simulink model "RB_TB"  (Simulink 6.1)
settings: Solver=ode3  SolverMode=SingleTasking  StartTime=0  StopTime=1000  FixedStep=0.05  RelTol=1e-3
libraries: simulink x2
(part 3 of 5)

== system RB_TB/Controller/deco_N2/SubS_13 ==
  note: Pt of seconds
  note: Model: RB_TB/Controller/deco_N2/SubS_X
  Palv : Inport  Port=1  LatchInput=off
  Pamb_sea : Inport  Port=2  LatchInput=off
  Palv_INI : Inport  Port=3  LatchInput=off
  HT : Inport  Port=4  LatchInput=off
  BC1 : BusCreator  DialogController=Simulink.DDGSource_Bus
  Mux6 : Mux  Inputs=3
  Product1 : Product
  Sum2 : Sum  Inputs=|+-
  Sum3 : Sum  Inputs=++|
  fcn3 : Fcn  Expr=u(3)+u(2)/u(1)
  fcn5 : Fcn  Expr=log(2)/u(1)
  fcn6 : Fcn  Expr=1.005-u(1)^(-1/2)
  fcn7 : Fcn  Expr=2*u(1)^(-1/3)
  pr_PN2 : TransferFcn  Numerator=[1/60]  Denominator=[1 0]
  bus : Outport
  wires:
  Sum2/1 -> Product1/2
  Product1/1 -> pr_PN2/1
  fcn3/1 -> BC1/4  "M0"
  fcn6/1 -> Mux6/1, BC1/3  "N2_b"
  Mux6/1 -> fcn3/1
  fcn5/1 -> Product1/1, BC1/1  "N2_k"
  Palv/1 -> Sum2/1
  Pamb_sea/1 -> Mux6/2
  fcn7/1 -> Mux6/3  "N2_a"
  Sum3/1 -> BC1/2, Sum2/2  "Pt"
  Palv_INI/1 -> Sum3/1
  pr_PN2/1 -> Sum3/2
  BC1/1 -> bus/1
  HT/1 -> fcn7/1, fcn5/1, fcn6/1

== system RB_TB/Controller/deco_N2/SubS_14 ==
  note: Model: RB_TB/Controller/deco_N2/SubS_X
  note: Pt of seconds
  Palv : Inport  Port=1  LatchInput=off
  Pamb_sea : Inport  Port=2  LatchInput=off
  Palv_INI : Inport  Port=3  LatchInput=off
  HT : Inport  Port=4  LatchInput=off
  BC1 : BusCreator  DialogController=Simulink.DDGSource_Bus
  Mux6 : Mux  Inputs=3
  Product1 : Product
  Sum2 : Sum  Inputs=|+-
  Sum3 : Sum  Inputs=++|
  fcn3 : Fcn  Expr=u(3)+u(2)/u(1)
  fcn5 : Fcn  Expr=log(2)/u(1)
  fcn6 : Fcn  Expr=1.005-u(1)^(-1/2)
  fcn7 : Fcn  Expr=2*u(1)^(-1/3)
  pr_PN2 : TransferFcn  Numerator=[1/60]  Denominator=[1 0]
  bus : Outport
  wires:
  HT/1 -> fcn6/1, fcn5/1, fcn7/1
  BC1/1 -> bus/1
  pr_PN2/1 -> Sum3/2
  Palv_INI/1 -> Sum3/1
  Sum3/1 -> Sum2/2, BC1/2  "Pt"
  fcn7/1 -> Mux6/3  "N2_a"
  Pamb_sea/1 -> Mux6/2
  Palv/1 -> Sum2/1
  fcn5/1 -> BC1/1, Product1/1  "N2_k"
  Mux6/1 -> fcn3/1
  fcn6/1 -> BC1/3, Mux6/1  "N2_b"
  fcn3/1 -> BC1/4  "M0"
  Product1/1 -> pr_PN2/1
  Sum2/1 -> Product1/2

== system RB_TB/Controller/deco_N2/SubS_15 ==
  note: Pt of seconds
  note: Model: RB_TB/Controller/deco_N2/SubS_X
  Palv : Inport  Port=1  LatchInput=off
  Pamb_sea : Inport  Port=2  LatchInput=off
  Palv_INI : Inport  Port=3  LatchInput=off
  HT : Inport  Port=4  LatchInput=off
  BC1 : BusCreator  DialogController=Simulink.DDGSource_Bus
  Mux6 : Mux  Inputs=3
  Product1 : Product
  Sum2 : Sum  Inputs=|+-
  Sum3 : Sum  Inputs=++|
  fcn3 : Fcn  Expr=u(3)+u(2)/u(1)
  fcn5 : Fcn  Expr=log(2)/u(1)
  fcn6 : Fcn  Expr=1.005-u(1)^(-1/2)
  fcn7 : Fcn  Expr=2*u(1)^(-1/3)
  pr_PN2 : TransferFcn  Numerator=[1/60]  Denominator=[1 0]
  bus : Outport
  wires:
  Sum2/1 -> Product1/2
  Product1/1 -> pr_PN2/1
  fcn3/1 -> BC1/4  "M0"
  fcn6/1 -> Mux6/1, BC1/3  "N2_b"
  Mux6/1 -> fcn3/1
  fcn5/1 -> Product1/1, BC1/1  "N2_k"
  Palv/1 -> Sum2/1
  Pamb_sea/1 -> Mux6/2
  fcn7/1 -> Mux6/3  "N2_a"
  Sum3/1 -> BC1/2, Sum2/2  "Pt"
  Palv_INI/1 -> Sum3/1
  pr_PN2/1 -> Sum3/2
  BC1/1 -> bus/1
  HT/1 -> fcn7/1, fcn5/1, fcn6/1

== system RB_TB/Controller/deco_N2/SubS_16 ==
  note: Model: RB_TB/Controller/deco_N2/SubS_X
  note: Pt of seconds
  Palv : Inport  Port=1  LatchInput=off
  Pamb_sea : Inport  Port=2  LatchInput=off
  Palv_INI : Inport  Port=3  LatchInput=off
  HT : Inport  Port=4  LatchInput=off
  BC1 : BusCreator  DialogController=Simulink.DDGSource_Bus
  Mux6 : Mux  Inputs=3
  Product1 : Product
  Sum2 : Sum  Inputs=|+-
  Sum3 : Sum  Inputs=++|
  fcn3 : Fcn  Expr=u(3)+u(2)/u(1)
  fcn5 : Fcn  Expr=log(2)/u(1)
  fcn6 : Fcn  Expr=1.005-u(1)^(-1/2)
  fcn7 : Fcn  Expr=2*u(1)^(-1/3)
  pr_PN2 : TransferFcn  Numerator=[1/60]  Denominator=[1 0]
  bus : Outport
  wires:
  HT/1 -> fcn6/1, fcn5/1, fcn7/1
  BC1/1 -> bus/1
  pr_PN2/1 -> Sum3/2
  Palv_INI/1 -> Sum3/1
  Sum3/1 -> Sum2/2, BC1/2  "Pt"
  fcn7/1 -> Mux6/3  "N2_a"
  Pamb_sea/1 -> Mux6/2
  Palv/1 -> Sum2/1
  fcn5/1 -> BC1/1, Product1/1  "N2_k"
  Mux6/1 -> fcn3/1
  fcn6/1 -> BC1/3, Mux6/1  "N2_b"
  fcn3/1 -> BC1/4  "M0"
  Product1/1 -> pr_PN2/1
  Sum2/1 -> Product1/2

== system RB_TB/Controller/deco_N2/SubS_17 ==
  note: Pt of seconds
  note: Model: RB_TB/Controller/deco_N2/SubS_X
  Palv : Inport  Port=1  LatchInput=off
  Pamb_sea : Inport  Port=2  LatchInput=off
  Palv_INI : Inport  Port=3  LatchInput=off
  HT : Inport  Port=4  LatchInput=off
  BC1 : BusCreator  DialogController=Simulink.DDGSource_Bus
  Mux6 : Mux  Inputs=3
  Product1 : Product
  Sum2 : Sum  Inputs=|+-
  Sum3 : Sum  Inputs=++|
  fcn3 : Fcn  Expr=u(3)+u(2)/u(1)
  fcn5 : Fcn  Expr=log(2)/u(1)
  fcn6 : Fcn  Expr=1.005-u(1)^(-1/2)
  fcn7 : Fcn  Expr=2*u(1)^(-1/3)
  pr_PN2 : TransferFcn  Numerator=[1/60]  Denominator=[1 0]
  bus : Outport
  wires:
  Sum2/1 -> Product1/2
  Product1/1 -> pr_PN2/1
  fcn3/1 -> BC1/4  "M0"
  fcn6/1 -> Mux6/1, BC1/3  "N2_b"
  Mux6/1 -> fcn3/1
  fcn5/1 -> Product1/1, BC1/1  "N2_k"
  Palv/1 -> Sum2/1
  Pamb_sea/1 -> Mux6/2
  fcn7/1 -> Mux6/3  "N2_a"
  Sum3/1 -> BC1/2, Sum2/2  "Pt"
  Palv_INI/1 -> Sum3/1
  pr_PN2/1 -> Sum3/2
  BC1/1 -> bus/1
  HT/1 -> fcn7/1, fcn5/1, fcn6/1

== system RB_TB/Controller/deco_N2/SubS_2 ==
  note: Model: RB_TB/Controller/deco_N2/SubS_X
  note: Pt of seconds
  Palv : Inport  Port=1  LatchInput=off
  Pamb_sea : Inport  Port=2  LatchInput=off
  Palv_INI : Inport  Port=3  LatchInput=off
  HT : Inport  Port=4  LatchInput=off
  BC1 : BusCreator  DialogController=Simulink.DDGSource_Bus
  Mux6 : Mux  Inputs=3
  Product1 : Product
  Sum2 : Sum  Inputs=|+-
  Sum3 : Sum  Inputs=++|
  fcn3 : Fcn  Expr=u(3)+u(2)/u(1)
  fcn5 : Fcn  Expr=log(2)/u(1)
  fcn6 : Fcn  Expr=1.005-u(1)^(-1/2)
  fcn7 : Fcn  Expr=2*u(1)^(-1/3)
  pr_PN2 : TransferFcn  Numerator=[1/60]  Denominator=[1 0]
  bus : Outport
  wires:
  HT/1 -> fcn6/1, fcn5/1, fcn7/1
  BC1/1 -> bus/1
  pr_PN2/1 -> Sum3/2
  Palv_INI/1 -> Sum3/1
  Sum3/1 -> Sum2/2, BC1/2  "Pt"
  fcn7/1 -> Mux6/3  "N2_a"
  Pamb_sea/1 -> Mux6/2
  Palv/1 -> Sum2/1
  fcn5/1 -> BC1/1, Product1/1  "N2_k"
  Mux6/1 -> fcn3/1
  fcn6/1 -> BC1/3, Mux6/1  "N2_b"
  fcn3/1 -> BC1/4  "M0"
  Product1/1 -> pr_PN2/1
  Sum2/1 -> Product1/2

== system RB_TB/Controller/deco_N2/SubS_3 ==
  note: Pt of seconds
  note: Model: RB_TB/Controller/deco_N2/SubS_X
  Palv : Inport  Port=1  LatchInput=off
  Pamb_sea : Inport  Port=2  LatchInput=off
  Palv_INI : Inport  Port=3  LatchInput=off
  HT : Inport  Port=4  LatchInput=off
  BC1 : BusCreator  DialogController=Simulink.DDGSource_Bus
  Mux6 : Mux  Inputs=3
  Product1 : Product
  Sum2 : Sum  Inputs=|+-
  Sum3 : Sum  Inputs=++|
  fcn3 : Fcn  Expr=u(3)+u(2)/u(1)
  fcn5 : Fcn  Expr=log(2)/u(1)
  fcn6 : Fcn  Expr=1.005-u(1)^(-1/2)
  fcn7 : Fcn  Expr=2*u(1)^(-1/3)
  pr_PN2 : TransferFcn  Numerator=[1/60]  Denominator=[1 0]
  bus : Outport
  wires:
  Sum2/1 -> Product1/2
  Product1/1 -> pr_PN2/1
  fcn3/1 -> BC1/4  "M0"
  fcn6/1 -> Mux6/1, BC1/3  "N2_b"
  Mux6/1 -> fcn3/1
  fcn5/1 -> Product1/1, BC1/1  "N2_k"
  Palv/1 -> Sum2/1
  Pamb_sea/1 -> Mux6/2
  fcn7/1 -> Mux6/3  "N2_a"
  Sum3/1 -> BC1/2, Sum2/2  "Pt"
  Palv_INI/1 -> Sum3/1
  pr_PN2/1 -> Sum3/2
  BC1/1 -> bus/1
  HT/1 -> fcn7/1, fcn5/1, fcn6/1

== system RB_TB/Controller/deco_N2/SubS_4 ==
  note: Model: RB_TB/Controller/deco_N2/SubS_X
  note: Pt of seconds
  Palv : Inport  Port=1  LatchInput=off
  Pamb_sea : Inport  Port=2  LatchInput=off
  Palv_INI : Inport  Port=3  LatchInput=off
  HT : Inport  Port=4  LatchInput=off
  BC1 : BusCreator  DialogController=Simulink.DDGSource_Bus
  Mux6 : Mux  Inputs=3
  Product1 : Product
  Sum2 : Sum  Inputs=|+-
  Sum3 : Sum  Inputs=++|
  fcn3 : Fcn  Expr=u(3)+u(2)/u(1)
  fcn5 : Fcn  Expr=log(2)/u(1)
  fcn6 : Fcn  Expr=1.005-u(1)^(-1/2)
  fcn7 : Fcn  Expr=2*u(1)^(-1/3)
  pr_PN2 : TransferFcn  Numerator=[1/60]  Denominator=[1 0]
  bus : Outport
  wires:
  HT/1 -> fcn6/1, fcn5/1, fcn7/1
  BC1/1 -> bus/1
  pr_PN2/1 -> Sum3/2
  Palv_INI/1 -> Sum3/1
  Sum3/1 -> Sum2/2, BC1/2  "Pt"
  fcn7/1 -> Mux6/3  "N2_a"
  Pamb_sea/1 -> Mux6/2
  Palv/1 -> Sum2/1
  fcn5/1 -> BC1/1, Product1/1  "N2_k"
  Mux6/1 -> fcn3/1
  fcn6/1 -> BC1/3, Mux6/1  "N2_b"
  fcn3/1 -> BC1/4  "M0"
  Product1/1 -> pr_PN2/1
  Sum2/1 -> Product1/2

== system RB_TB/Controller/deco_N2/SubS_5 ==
  note: Pt of seconds
  note: Model: RB_TB/Controller/deco_N2/SubS_X
  Palv : Inport  Port=1  LatchInput=off
  Pamb_sea : Inport  Port=2  LatchInput=off
  Palv_INI : Inport  Port=3  LatchInput=off
  HT : Inport  Port=4  LatchInput=off
  BC1 : BusCreator  DialogController=Simulink.DDGSource_Bus
  Mux6 : Mux  Inputs=3
  Product1 : Product
  Sum2 : Sum  Inputs=|+-
  Sum3 : Sum  Inputs=++|
  fcn3 : Fcn  Expr=u(3)+u(2)/u(1)
  fcn5 : Fcn  Expr=log(2)/u(1)
  fcn6 : Fcn  Expr=1.005-u(1)^(-1/2)
  fcn7 : Fcn  Expr=2*u(1)^(-1/3)
  pr_PN2 : TransferFcn  Numerator=[1/60]  Denominator=[1 0]
  bus : Outport
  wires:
  Sum2/1 -> Product1/2
  Product1/1 -> pr_PN2/1
  fcn3/1 -> BC1/4  "M0"
  fcn6/1 -> Mux6/1, BC1/3  "N2_b"
  Mux6/1 -> fcn3/1
  fcn5/1 -> Product1/1, BC1/1  "N2_k"
  Palv/1 -> Sum2/1
  Pamb_sea/1 -> Mux6/2
  fcn7/1 -> Mux6/3  "N2_a"
  Sum3/1 -> BC1/2, Sum2/2  "Pt"
  Palv_INI/1 -> Sum3/1
  pr_PN2/1 -> Sum3/2
  BC1/1 -> bus/1
  HT/1 -> fcn7/1, fcn5/1, fcn6/1

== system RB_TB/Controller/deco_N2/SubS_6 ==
  note: Model: RB_TB/Controller/deco_N2/SubS_X
  note: Pt of seconds
  Palv : Inport  Port=1  LatchInput=off
  Pamb_sea : Inport  Port=2  LatchInput=off
  Palv_INI : Inport  Port=3  LatchInput=off
  HT : Inport  Port=4  LatchInput=off
  BC1 : BusCreator  DialogController=Simulink.DDGSource_Bus
  Mux6 : Mux  Inputs=3
  Product1 : Product
  Sum2 : Sum  Inputs=|+-
  Sum3 : Sum  Inputs=++|
  fcn3 : Fcn  Expr=u(3)+u(2)/u(1)
  fcn5 : Fcn  Expr=log(2)/u(1)
  fcn6 : Fcn  Expr=1.005-u(1)^(-1/2)
  fcn7 : Fcn  Expr=2*u(1)^(-1/3)
  pr_PN2 : TransferFcn  Numerator=[1/60]  Denominator=[1 0]
  bus : Outport
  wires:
  HT/1 -> fcn6/1, fcn5/1, fcn7/1
  BC1/1 -> bus/1
  pr_PN2/1 -> Sum3/2
  Palv_INI/1 -> Sum3/1
  Sum3/1 -> Sum2/2, BC1/2  "Pt"
  fcn7/1 -> Mux6/3  "N2_a"
  Pamb_sea/1 -> Mux6/2
  Palv/1 -> Sum2/1
  fcn5/1 -> BC1/1, Product1/1  "N2_k"
  Mux6/1 -> fcn3/1
  fcn6/1 -> BC1/3, Mux6/1  "N2_b"
  fcn3/1 -> BC1/4  "M0"
  Product1/1 -> pr_PN2/1
  Sum2/1 -> Product1/2

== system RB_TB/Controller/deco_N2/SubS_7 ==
  note: Pt of seconds
  note: Model: RB_TB/Controller/deco_N2/SubS_X
  Palv : Inport  Port=1  LatchInput=off
  Pamb_sea : Inport  Port=2  LatchInput=off
  Palv_INI : Inport  Port=3  LatchInput=off
  HT : Inport  Port=4  LatchInput=off
  BC1 : BusCreator  DialogController=Simulink.DDGSource_Bus
  Mux6 : Mux  Inputs=3
  Product1 : Product
  Sum2 : Sum  Inputs=|+-
  Sum3 : Sum  Inputs=++|
  fcn3 : Fcn  Expr=u(3)+u(2)/u(1)
  fcn5 : Fcn  Expr=log(2)/u(1)
  fcn6 : Fcn  Expr=1.005-u(1)^(-1/2)
  fcn7 : Fcn  Expr=2*u(1)^(-1/3)
  pr_PN2 : TransferFcn  Numerator=[1/60]  Denominator=[1 0]
  bus : Outport
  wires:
  Sum2/1 -> Product1/2
  Product1/1 -> pr_PN2/1
  fcn3/1 -> BC1/4  "M0"
  fcn6/1 -> Mux6/1, BC1/3  "N2_b"
  Mux6/1 -> fcn3/1
  fcn5/1 -> Product1/1, BC1/1  "N2_k"
  Palv/1 -> Sum2/1
  Pamb_sea/1 -> Mux6/2
  fcn7/1 -> Mux6/3  "N2_a"
  Sum3/1 -> BC1/2, Sum2/2  "Pt"
  Palv_INI/1 -> Sum3/1
  pr_PN2/1 -> Sum3/2
  BC1/1 -> bus/1
  HT/1 -> fcn7/1, fcn5/1, fcn6/1

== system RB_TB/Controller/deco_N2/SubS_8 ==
  note: Model: RB_TB/Controller/deco_N2/SubS_X
  note: Pt of seconds
  Palv : Inport  Port=1  LatchInput=off
  Pamb_sea : Inport  Port=2  LatchInput=off
  Palv_INI : Inport  Port=3  LatchInput=off
  HT : Inport  Port=4  LatchInput=off
  BC1 : BusCreator  DialogController=Simulink.DDGSource_Bus
  Mux6 : Mux  Inputs=3
  Product1 : Product
  Sum2 : Sum  Inputs=|+-
  Sum3 : Sum  Inputs=++|
  fcn3 : Fcn  Expr=u(3)+u(2)/u(1)
  fcn5 : Fcn  Expr=log(2)/u(1)
  fcn6 : Fcn  Expr=1.005-u(1)^(-1/2)
  fcn7 : Fcn  Expr=2*u(1)^(-1/3)
  pr_PN2 : TransferFcn  Numerator=[1/60]  Denominator=[1 0]
  bus : Outport
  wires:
  HT/1 -> fcn6/1, fcn5/1, fcn7/1
  BC1/1 -> bus/1
  pr_PN2/1 -> Sum3/2
  Palv_INI/1 -> Sum3/1
  Sum3/1 -> Sum2/2, BC1/2  "Pt"
  fcn7/1 -> Mux6/3  "N2_a"
  Pamb_sea/1 -> Mux6/2
  Palv/1 -> Sum2/1
  fcn5/1 -> BC1/1, Product1/1  "N2_k"
  Mux6/1 -> fcn3/1
  fcn6/1 -> BC1/3, Mux6/1  "N2_b"
  fcn3/1 -> BC1/4  "M0"
  Product1/1 -> pr_PN2/1
  Sum2/1 -> Product1/2

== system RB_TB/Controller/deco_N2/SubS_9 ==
  note: Pt of seconds
  note: Model: RB_TB/Controller/deco_N2/SubS_X
  Palv : Inport  Port=1  LatchInput=off
  Pamb_sea : Inport  Port=2  LatchInput=off
  Palv_INI : Inport  Port=3  LatchInput=off
  HT : Inport  Port=4  LatchInput=off
  BC1 : BusCreator  DialogController=Simulink.DDGSource_Bus
  Mux6 : Mux  Inputs=3
  Product1 : Product
  Sum2 : Sum  Inputs=|+-
  Sum3 : Sum  Inputs=++|
  fcn3 : Fcn  Expr=u(3)+u(2)/u(1)
  fcn5 : Fcn  Expr=log(2)/u(1)
  fcn6 : Fcn  Expr=1.005-u(1)^(-1/2)
  fcn7 : Fcn  Expr=2*u(1)^(-1/3)
  pr_PN2 : TransferFcn  Numerator=[1/60]  Denominator=[1 0]
  bus : Outport
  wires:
  Sum2/1 -> Product1/2
  Product1/1 -> pr_PN2/1
  fcn3/1 -> BC1/4  "M0"
  fcn6/1 -> Mux6/1, BC1/3  "N2_b"
  Mux6/1 -> fcn3/1
  fcn5/1 -> Product1/1, BC1/1  "N2_k"
  Palv/1 -> Sum2/1
  Pamb_sea/1 -> Mux6/2
  fcn7/1 -> Mux6/3  "N2_a"
  Sum3/1 -> BC1/2, Sum2/2  "Pt"
  Palv_INI/1 -> Sum3/1
  pr_PN2/1 -> Sum3/2
  BC1/1 -> bus/1
  HT/1 -> fcn7/1, fcn5/1, fcn6/1

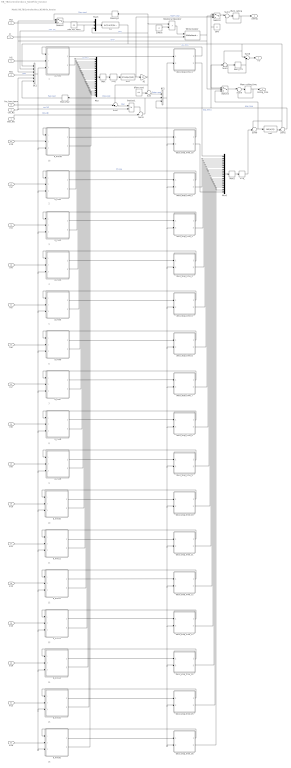
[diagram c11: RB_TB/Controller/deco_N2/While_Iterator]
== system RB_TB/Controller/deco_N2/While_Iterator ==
  note: 1
  note: 2
  note: 3
  note: 4
  note: 5
  note: 6
  note: 7
  note: 8
  note: 9
  note: 10
  note: 11
  note: 12
  note: 13
  note: 14
  note: 15
  note: 16
  note: Model: RB_TB/Controller/deco_N2/While_Iterator
  note: 1b
  cnc_N2 : Inport  Port=1  LatchInput=off
  Psw : Inport  Port=2  LatchInput=off
  IC : Inport  Port=3  LatchInput=off
  Palv : Inport  Port=4  LatchInput=off
  In1 : Inport  Port=5  LatchInput=off
  In2 : Inport  Port=6  LatchInput=off
  Palv_INI : Inport  Port=7  LatchInput=off
  fnc_hum_temp : Inport  Port=8  LatchInput=off
  In3 : Inport  Port=9  LatchInput=off
  In4 : Inport  Port=10  LatchInput=off
  In5 : Inport  Port=11  LatchInput=off
  In6 : Inport  Port=12  LatchInput=off
  In7 : Inport  Port=13  LatchInput=off
  In8 : Inport  Port=14  LatchInput=off
  In9 : Inport  Port=15  LatchInput=off
  In10 : Inport  Port=16  LatchInput=off
  In11 : Inport  Port=17  LatchInput=off
  In12 : Inport  Port=18  LatchInput=off
  In13 : Inport  Port=19  LatchInput=off
  In14 : Inport  Port=20  LatchInput=off
  In15 : Inport  Port=21  LatchInput=off
  In16 : Inport  Port=22  LatchInput=off
  In1b : Inport  Port=23  LatchInput=off
  >=0 : DeadZone  LowerValue=-1000  UpperValue=0
  >=0_ : DeadZone  LowerValue=-inf  UpperValue=0
  BC1 : BusCreator  DialogController=Simulink.DDGSource_Bus  Inputs=6
  BC2 : BusCreator  DialogController=Simulink.DDGSource_Bus  Inputs=3
  K1 : Gain  Gain=0.1
  Max : MinMax  Function=max
  Max1 : MinMax  Function=max
  Mem_Palv : Memory  Orientation=left  InheritSampleTime=on
  Mem_TTS : Memory  InheritSampleTime=on
  Mem_ceiling : Memory  InheritSampleTime=on
  Mem_ceiling_time : Memory  InheritSampleTime=on
  Memory2 : Memory  Orientation=left  InheritSampleTime=on
  Mux : Mux  Inputs=17
  Mux1 : Mux  Inputs=17
  Mux3 : Mux  Inputs=3
  Product1 : Product
  Relational Operator : RelationalOperator  Operator=>  LogicOutDataTypeMode=Boolean
  Suface : Constant  Value=0
  Sum : Sum  Inputs=+-|
  Sum1 : Sum  Inputs=|++
  Sum2 : Sum  Inputs=-+|
  Sum3 : Sum  Inputs=+++
  Sum4 : Sum  Inputs=|++
  Sum5 : Sum
  Sum6 : Sum  Inputs=++|
  Sum7 : Sum  Inputs=++|
  Sum8 : Sum
  Switch1 : Switch  Threshold=2
  Switch2 : Switch  Threshold=2
  Switch3 : Switch  Threshold=2
  While Iterator : WhileIterator  MaxIters=100  ShowIterationPort=on
  dPsw_next : Constant  Value=0.3
  d_min1 : Subsystem
  d_min10 : Subsystem
  d_min11 : Subsystem
  d_min12 : Subsystem
  d_min13 : Subsystem
  d_min14 : Subsystem
  d_min15 : Subsystem
  d_min16 : Subsystem
  d_min1b : Subsystem
  d_min2 : Subsystem
  d_min3 : Subsystem
  d_min4 : Subsystem
  d_min5 : Subsystem
  d_min6 : Subsystem
  d_min7 : Subsystem
  d_min8 : Subsystem
  d_min9 : Subsystem
  deco_stop_time_1 : Subsystem
  deco_stop_time_10 : Subsystem
  deco_stop_time_11 : Subsystem
  deco_stop_time_12 : Subsystem
  deco_stop_time_13 : Subsystem
  deco_stop_time_14 : Subsystem
  deco_stop_time_15 : Subsystem
  deco_stop_time_16 : Subsystem
  deco_stop_time_1b : Subsystem
  deco_stop_time_2 : Subsystem
  deco_stop_time_3 : Subsystem
  deco_stop_time_4 : Subsystem
  deco_stop_time_5 : Subsystem
  deco_stop_time_6 : Subsystem
  deco_stop_time_7 : Subsystem
  deco_stop_time_8 : Subsystem
  deco_stop_time_9 : Subsystem
  fcn : Fcn  Expr=(u(1)-u(3))/u(2)
  fcn1 : Fcn  Expr=ceil(u(1))
  fcn2 : Fcn  Expr=3*ceil(u(1)/3)
  rate_asc_deco : Constant  Value=0.9
  zero : Constant  Orientation=left  Value=0
  TTS : Outport
  ceiling : Outport  Port=2
  ceiling_time : Outport  Port=3
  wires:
  IC/1 -> While Iterator/2
  Mux/1 -> Max/1
  fcn2/1 -> K1/1, Switch1/3  "Depth_stop"
  Max/1 -> >=0/1
  >=0/1 -> fcn2/1
  rate_asc_deco/1 -> Mux3/2, BC1/2  "rate_asc"
  K1/1 -> Sum7/1, Sum/1, Mux3/3, Memory2/1, Relational Operator/1  "Psw"
  Max1/1 -> >=0_/1
  Mux3/1 -> fcn/1
  deco_stop_time_1/2(deco_stop_time) -> Mux1/1  "stop_time_i"
  fcn/1 -> Sum8/1, Sum3/1, Sum2/1, Sum6/1, BC1/1  "asc_time"
  d_min1/2(d_min) -> Mux/1  "d_min_i"
  Mem_TTS/1 -> Sum8/2, Sum3/3
  Sum3/1 -> Mem_TTS/1
  cnc_N2/1 -> Product1/2, BC1/5  "cnc_N2"
  Product1/1 -> Sum5/1
  Palv_INI/1 -> Sum5/2  "Palv_INI"
  fnc_hum_temp/1 -> Sum7/2
  Sum5/1 -> Mem_Palv/1, BC2/2  "Palv_next"
  Sum7/1 -> Product1/1  "Psw'"
  d_min1/1(bus1) -> deco_stop_time_1/1(bus1)
  d_min2/1(bus1) -> deco_stop_time_2/1(bus1)
  d_min2/2(d_min) -> Mux/2
  In1/1 -> d_min1/2(In1)
  Mem_Palv/1 -> BC1/6  "Palv_next"
  Psw/1 -> Switch2/3
  Switch2/1 -> Mux3/1
  Memory2/1 -> Switch2/1  "Psw_nwxt"
  deco_stop_time_1/1(Pt_new) -> d_min1/1(Pt_new)
  dPsw_next/1 -> Sum/2
  Sum/1 -> BC2/1  "Pstop_next"
  deco_stop_time_2/1(Pt_new) -> d_min2/1(Pt_new)  "Pt_new"
  Sum2/1 -> BC2/3, Sum3/2  "stop_time"
  fcn1/1 -> Sum2/2
  Sum6/1 -> fcn1/1, Switch3/3
  >=0_/1 -> Sum6/2
  Suface/1 -> Relational Operator/2
  Relational Operator/1 -> While Iterator/1
  Sum1/1 -> Mem_ceiling/1
  Mem_ceiling/1 -> ceiling/1, Sum1/2
  Switch1/1 -> Sum1/1
  Mem_ceiling_time/1 -> ceiling_time/1, Sum4/2
  Sum8/1 -> TTS/1
  Palv/1 -> BC1/4  "Palv"
  BC1/1 -> d_min1/3(In2), d_min15/3(In2), d_min16/3(In2), d_min14/3(In2), d_min13/3(In2), d_min12/3(In2), d_min11/3(In2), d_min10/3(In2), d_min9/3(In2), d_min8/3(In2), d_min7/3(In2), d_min6/3(In2), d_min5/3(In2), d_min4/3(In2), d_min3/3(In2), d_min2/3(In2), d_min1b/3(In2)
  In2/1 -> d_min2/2(In1)
  BC2/1 -> deco_stop_time_1/2(bus2), deco_stop_time_15/2(bus2), deco_stop_time_16/2(bus2), deco_stop_time_14/2(bus2), deco_stop_time_13/2(bus2), deco_stop_time_12/2(bus2), deco_stop_time_11/2(bus2), deco_stop_time_10/2(bus2), deco_stop_time_9/2(bus2), deco_stop_time_8/2(bus2), deco_stop_time_7/2(bus2), deco_stop_time_6/2(bus2), deco_stop_time_5/2(bus2), deco_stop_time_4/2(bus2), deco_stop_time_3/2(bus2), deco_stop_time_2/2(bus2), deco_stop_time_1b/2(bus2)
  zero/1 -> Switch1/1, Switch3/1
  While Iterator/1 -> BC1/3, Switch2/2, Switch3/2, Switch1/2  "while"
  d_min3/1(bus1) -> deco_stop_time_3/1(bus1)
  deco_stop_time_3/1(Pt_new) -> d_min3/1(Pt_new)
  In3/1 -> d_min3/2(In1)
  In4/1 -> d_min4/2(In1)
  deco_stop_time_4/1(Pt_new) -> d_min4/1(Pt_new)
  d_min4/1(bus1) -> deco_stop_time_4/1(bus1)
  d_min5/1(bus1) -> deco_stop_time_5/1(bus1)
  deco_stop_time_5/1(Pt_new) -> d_min5/1(Pt_new)
  In5/1 -> d_min5/2(In1)
  In6/1 -> d_min6/2(In1)
  deco_stop_time_6/1(Pt_new) -> d_min6/1(Pt_new)
  d_min6/1(bus1) -> deco_stop_time_6/1(bus1)
  d_min7/1(bus1) -> deco_stop_time_7/1(bus1)
  deco_stop_time_7/1(Pt_new) -> d_min7/1(Pt_new)
  In7/1 -> d_min7/2(In1)
  In8/1 -> d_min8/2(In1)
  deco_stop_time_8/1(Pt_new) -> d_min8/1(Pt_new)
  d_min8/1(bus1) -> deco_stop_time_8/1(bus1)
  d_min9/1(bus1) -> deco_stop_time_9/1(bus1)
  deco_stop_time_9/1(Pt_new) -> d_min9/1(Pt_new)
  In9/1 -> d_min9/2(In1)
  In10/1 -> d_min10/2(In1)
  deco_stop_time_10/1(Pt_new) -> d_min10/1(Pt_new)
  d_min10/1(bus1) -> deco_stop_time_10/1(bus1)
  d_min11/1(bus1) -> deco_stop_time_11/1(bus1)
  deco_stop_time_11/1(Pt_new) -> d_min11/1(Pt_new)
  In11/1 -> d_min11/2(In1)
  In12/1 -> d_min12/2(In1)
  deco_stop_time_12/1(Pt_new) -> d_min12/1(Pt_new)
  d_min12/1(bus1) -> deco_stop_time_12/1(bus1)
  d_min13/1(bus1) -> deco_stop_time_13/1(bus1)
  deco_stop_time_13/1(Pt_new) -> d_min13/1(Pt_new)
  In13/1 -> d_min13/2(In1)
  In14/1 -> d_min14/2(In1)
  deco_stop_time_14/1(Pt_new) -> d_min14/1(Pt_new)
  d_min14/1(bus1) -> deco_stop_time_14/1(bus1)
  d_min15/1(bus1) -> deco_stop_time_15/1(bus1)
  deco_stop_time_15/1(Pt_new) -> d_min15/1(Pt_new)
  In15/1 -> d_min15/2(In1)
  In16/1 -> d_min16/2(In1)
  deco_stop_time_16/1(Pt_new) -> d_min16/1(Pt_new)
  d_min16/1(bus1) -> deco_stop_time_16/1(bus1)
  Mux1/1 -> Max1/1
  deco_stop_time_2/2(deco_stop_time) -> Mux1/2
  d_min3/2(d_min) -> Mux/3
  d_min4/2(d_min) -> Mux/4
  d_min5/2(d_min) -> Mux/5
  d_min6/2(d_min) -> Mux/6
  d_min7/2(d_min) -> Mux/7
  d_min8/2(d_min) -> Mux/8
  d_min9/2(d_min) -> Mux/9
  d_min10/2(d_min) -> Mux/10
  d_min11/2(d_min) -> Mux/11
  d_min12/2(d_min) -> Mux/12
  d_min13/2(d_min) -> Mux/13
  d_min14/2(d_min) -> Mux/14
  d_min15/2(d_min) -> Mux/15
  d_min16/2(d_min) -> Mux/16
  deco_stop_time_3/2(deco_stop_time) -> Mux1/3
  deco_stop_time_4/2(deco_stop_time) -> Mux1/4
  deco_stop_time_5/2(deco_stop_time) -> Mux1/5
  deco_stop_time_6/2(deco_stop_time) -> Mux1/6
  deco_stop_time_7/2(deco_stop_time) -> Mux1/7
  deco_stop_time_8/2(deco_stop_time) -> Mux1/8
  deco_stop_time_9/2(deco_stop_time) -> Mux1/9
  deco_stop_time_10/2(deco_stop_time) -> Mux1/10
  deco_stop_time_11/2(deco_stop_time) -> Mux1/11
  deco_stop_time_12/2(deco_stop_time) -> Mux1/12
  deco_stop_time_13/2(deco_stop_time) -> Mux1/13
  deco_stop_time_14/2(deco_stop_time) -> Mux1/14
  deco_stop_time_15/2(deco_stop_time) -> Mux1/15
  deco_stop_time_16/2(deco_stop_time) -> Mux1/16
  Sum4/1 -> Mem_ceiling_time/1
  Switch3/1 -> Sum4/1
  d_min1b/1(bus1) -> deco_stop_time_1b/1(bus1)
  deco_stop_time_1b/1(Pt_new) -> d_min1b/1(Pt_new)
  In1b/1 -> d_min1b/2(In1)
  d_min1b/2(d_min) -> Mux/17
  deco_stop_time_1b/2(deco_stop_time) -> Mux1/17

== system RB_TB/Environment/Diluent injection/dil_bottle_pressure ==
  note: Model: RB_TB/Environment/Diluent injection/pr_dil_bottle
  gas_mix : Inport  Port=1  LatchInput=off
  F_D : Inport  Port=2  LatchInput=off
  Fcn : Fcn  Expr=u(1)/u(2)
  Multiport Switch : MultiPortSwitch  Inputs=3
  Multiport Switch1 : MultiPortSwitch  Inputs=3
  Multiport Switch2 : MultiPortSwitch  Inputs=3
  Mux : Mux  Inputs=2
  Product : Product
  Product2 : Product
  Product3 : Product
  Sum : Sum  Inputs=+-
  Sum2 : Sum  Inputs=+-
  Sum3 : Sum  Inputs=+-
  Sw1 : MultiPortSwitch  Inputs=3
  Sw3 : MultiPortSwitch  Inputs=3
  Sw4 : MultiPortSwitch  Inputs=3
  integral1 : Integrator
  integral2 : Integrator
  integral3 : Integrator
  pr_dil_bottle1_ini : Constant  Value=230
  pr_dil_bottle2_ini : Constant  Value=230
  pr_dil_bottle3_ini : Constant  Value=230
  size_dil_bottle1 : Constant  Value=3
  size_dil_bottle2 : Constant  Value=3
  size_dil_bottle3 : Constant  Value=3
  zero : Constant  Value=0
  O2 : Outport
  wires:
  Product/1 -> Sum/1  "vol_dil_bottle1_ini"
  integral1/1 -> Sum/2
  gas_mix/1 -> Sw4/1, Sw3/1, Sw1/1, Multiport Switch/1, Multiport Switch1/1, Multiport Switch2/1
  Sum/1 -> Multiport Switch/2
  Multiport Switch/1 -> Mux/1  "vol_dil_bottle"
  Sw1/1 -> integral1/1
  zero/1 -> Sw4/4, Sw3/2, Sw3/3, Sw4/2, Sw1/3, Sw1/4
  F_D/1 -> Sw1/2, Sw4/3, Sw3/4
  Mux/1 -> Fcn/1
  Fcn/1 -> O2/1  "pr_dil_bottle"
  size_dil_bottle1/1 -> Product/1, Multiport Switch1/2
  pr_dil_bottle1_ini/1 -> Product/2, Multiport Switch2/2
  Product2/1 -> Sum2/1  "vol_dil_bottle2_ini"
  integral2/1 -> Sum2/2
  Sw4/1 -> integral2/1
  size_dil_bottle2/1 -> Product2/1, Multiport Switch1/3
  pr_dil_bottle2_ini/1 -> Product2/2, Multiport Switch2/3
  Product3/1 -> Sum3/1  "vol_dil_bottle3_ini"
  integral3/1 -> Sum3/2
  Sw3/1 -> integral3/1
  size_dil_bottle3/1 -> Product3/1, Multiport Switch1/4
  pr_dil_bottle3_ini/1 -> Product3/2, Multiport Switch2/4
  Sum2/1 -> Multiport Switch/3
  Sum3/1 -> Multiport Switch/4
  Multiport Switch1/1 -> Mux/2  "size_dil_bottle"
  Multiport Switch2/1 -> [pr_dil_bottle_ini]

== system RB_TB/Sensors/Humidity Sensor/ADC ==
  note: Model: RB_TB/Sensors/Humidity_sensor/ADC
  note: This subsystem models a typical 16-bit analog-to-digital converter having an input range of 0-5 volts
  voltage : Inport  Port=1  LatchInput=off
  limit : Saturate  UpperLimit=65535  LowerLimit=0
  quantize : Quantizer  QuantizationInterval=1
  scale : Gain  Gain=65536/5
  pcm : Outport
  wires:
  limit/1 -> pcm/1
  scale/1 -> quantize/1
  quantize/1 -> limit/1
  voltage/1 -> scale/1

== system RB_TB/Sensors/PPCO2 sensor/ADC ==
  note: This subsystem models a typical 16-bit analog-to-digital converter having an input range of 0-5 volts
  note: Model: RB_TB/Sensors/PPCO2 sensor/ADC
  voltage : Inport  Port=1  LatchInput=off
  limit : Saturate  UpperLimit=65535  LowerLimit=0
  quantize : Quantizer  QuantizationInterval=1
  scale : Gain  Gain=65536/5
  pcm : Outport
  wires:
  voltage/1 -> scale/1
  quantize/1 -> limit/1
  scale/1 -> quantize/1
  limit/1 -> pcm/1

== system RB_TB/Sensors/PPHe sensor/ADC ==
  note: Model: RB_TB/Sensors/PPO2 sensor/ADC
  note: This subsystem models a typical 16-bit analog-to-digital converter having an input range of 0-5 volts
  voltage : Inport  Port=1  LatchInput=off
  limit : Saturate  UpperLimit=65535  LowerLimit=0
  quantize : Quantizer  QuantizationInterval=1
  scale : Gain  Gain=65536/5
  pcm : Outport
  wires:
  voltage/1 -> scale/1
  quantize/1 -> limit/1
  scale/1 -> quantize/1
  limit/1 -> pcm/1

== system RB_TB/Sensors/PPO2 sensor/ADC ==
  note: This subsystem models a typical 16-bit analog-to-digital converter having an input range of 0-5 volts
  note: Model: RB_TB/Sensors/PPO2 sensor/ADC
  voltage : Inport  Port=1  LatchInput=off
  limit : Saturate  UpperLimit=65535  LowerLimit=0
  quantize : Quantizer  QuantizationInterval=1
  scale : Gain  Gain=65536/5
  pcm : Outport
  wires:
  limit/1 -> pcm/1
  scale/1 -> quantize/1
  quantize/1 -> limit/1
  voltage/1 -> scale/1

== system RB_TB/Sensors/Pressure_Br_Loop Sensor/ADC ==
  note: This subsystem models a typical 15-bit analog-to-digital converter having an input range of 0-3 volts
  note: Model: RB_TB/Sensors/Pressure_ambient Sensor/ADC
  voltage : Inport  Port=1  LatchInput=off
  limit : Saturate  UpperLimit=2^15  LowerLimit=0
  quantize : Quantizer  QuantizationInterval=1
  scale : Gain  Gain=2^15/3
  pcm : Outport
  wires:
  voltage/1 -> scale/1
  quantize/1 -> limit/1
  scale/1 -> quantize/1
  limit/1 -> pcm/1

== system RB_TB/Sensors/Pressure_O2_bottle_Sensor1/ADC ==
  note: Model: RB_TB/Sensors/Pressure_ambient Sensor/ADC
  note: This subsystem models a typical 15-bit analog-to-digital converter having an input range of 0-3 volts
  voltage : Inport  Port=1  LatchInput=off
  limit : Saturate  UpperLimit=2^15  LowerLimit=0
  quantize : Quantizer  QuantizationInterval=1
  scale : Gain  Gain=2^15/3
  pcm : Outport
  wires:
  limit/1 -> pcm/1
  scale/1 -> quantize/1
  quantize/1 -> limit/1
  voltage/1 -> scale/1

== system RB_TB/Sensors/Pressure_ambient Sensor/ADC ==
  note: Model: RB_TB/Sensors/Pressure_ambient Sensor/ADC
  note: This subsystem models a typical 15-bit analog-to-digital converter having an input range of 0-3 volts
  voltage : Inport  Port=1  LatchInput=off
  limit : Saturate  UpperLimit=2^15  LowerLimit=0
  quantize : Quantizer  QuantizationInterval=1
  scale : Gain  Gain=2^15/3
  pcm : Outport
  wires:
  limit/1 -> pcm/1
  scale/1 -> quantize/1
  quantize/1 -> limit/1
  voltage/1 -> scale/1

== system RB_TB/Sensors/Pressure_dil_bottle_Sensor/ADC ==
  note: This subsystem models a typical 15-bit analog-to-digital converter having an input range of 0-3 volts
  note: Model: RB_TB/Sensors/Pressure_ambient Sensor/ADC
  voltage : Inport  Port=1  LatchInput=off
  limit : Saturate  UpperLimit=2^15  LowerLimit=0
  quantize : Quantizer  QuantizationInterval=1
  scale : Gain  Gain=2^15/3
  pcm : Outport
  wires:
  voltage/1 -> scale/1
  quantize/1 -> limit/1
  scale/1 -> quantize/1
  limit/1 -> pcm/1

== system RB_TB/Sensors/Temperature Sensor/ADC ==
  note: This subsystem models a typical 16-bit analog-to-digital converter having an input range of 0-5 volts
  note: Model: RB_TB/Sensors/temperature_sensor/ADC
  voltage : Inport  Port=1  LatchInput=off
  limit : Saturate  UpperLimit=65535  LowerLimit=0
  quantize : Quantizer  QuantizationInterval=1
  scale : Gain  Gain=65536/5
  pcm : Outport
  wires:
  voltage/1 -> scale/1
  quantize/1 -> limit/1
  scale/1 -> quantize/1
  limit/1 -> pcm/1

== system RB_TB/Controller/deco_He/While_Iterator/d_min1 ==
  note: Model: RB_TB/Controller/deco_He/While_Iterator/d_minX
  Pt_new : Inport  Port=1  LatchInput=off
  In1 : Inport  Port=2  LatchInput=off
  In2 : Inport  Port=3  LatchInput=off
  BC : BusCreator  DialogController=Simulink.DDGSource_Bus
  BS1 : BusSelector  DialogController=Simulink.DDGSource_Bus  OutputSignals=He_b,M0,He_k,Pt
  BS2 : BusSelector  DialogController=Simulink.DDGSource_Bus  OutputSignals=rate_asc,asc_time,while,cnc_He,Palv_next,Palv
  Mux2 : Mux  Inputs=6
  Product2 : Product
  Sum1 : Sum  Inputs=-+|
  Switch : Switch  Threshold=2
  Switch1 : Switch  Threshold=2
  fnc : Fcn  Expr=u(6)-u(5)*u(2)*(u(3)-1/u(1))-(u(6)-u(4)+u(5)*u(2)/u(1))*exp(-u(1)*u(3))
  prod : Gain  Gain=10
  bus1 : Outport
  d_min : Outport  Port=2
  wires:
  BS2/1 -> Mux2/2  "<rate_asc>"
  In2/1 -> BS2/1
  BS2/5 -> Switch1/1  "<Palv_next>"
  BS2/3 -> Switch1/2, Switch/2  "<while>"
  BS2/6 -> Switch1/3  "<Palv>"
  Switch1/1 -> Mux2/6
  Pt_new/1 -> Switch/1
  BS1/4 -> Switch/3  "<Pt>"
  Switch/1 -> Mux2/4, Sum1/2  "Pt"
  BC/1 -> bus1/1
  Product2/1 -> d_min/1
  prod/1 -> Product2/1
  Sum1/1 -> Product2/2
  In1/1 -> BS1/1
  BS2/4 -> Mux2/5  "<cnc_He>"
  BS2/2 -> Mux2/3  "<asc_time>"
  fnc/1 -> BC/4  "Pt_stop"
  Mux2/1 -> fnc/1
  BS1/2 -> BC/2, Sum1/1  "<M0>"
  BS1/1 -> BC/1, prod/1  "<He_b>"
  BS1/3 -> BC/3, Mux2/1  "<He_k>"

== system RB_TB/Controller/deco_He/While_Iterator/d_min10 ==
  note: Model: RB_TB/Controller/deco_He/While_Iterator/d_minX
  Pt_new : Inport  Port=1  LatchInput=off
  In1 : Inport  Port=2  LatchInput=off
  In2 : Inport  Port=3  LatchInput=off
  BC : BusCreator  DialogController=Simulink.DDGSource_Bus
  BS1 : BusSelector  DialogController=Simulink.DDGSource_Bus  OutputSignals=He_b,M0,He_k,Pt
  BS2 : BusSelector  DialogController=Simulink.DDGSource_Bus  OutputSignals=rate_asc,asc_time,while,cnc_He,Palv_next,Palv
  Mux2 : Mux  Inputs=6
  Product2 : Product
  Sum1 : Sum  Inputs=-+|
  Switch : Switch  Threshold=2
  Switch1 : Switch  Threshold=2
  fnc : Fcn  Expr=u(6)-u(5)*u(2)*(u(3)-1/u(1))-(u(6)-u(4)+u(5)*u(2)/u(1))*exp(-u(1)*u(3))
  prod : Gain  Gain=10
  bus1 : Outport
  d_min : Outport  Port=2
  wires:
  BS1/3 -> Mux2/1, BC/3  "<He_k>"
  BS1/1 -> prod/1, BC/1  "<He_b>"
  BS1/2 -> Sum1/1, BC/2  "<M0>"
  Mux2/1 -> fnc/1
  fnc/1 -> BC/4  "Pt_stop"
  BS2/2 -> Mux2/3  "<asc_time>"
  BS2/4 -> Mux2/5  "<cnc_He>"
  In1/1 -> BS1/1
  Sum1/1 -> Product2/2
  prod/1 -> Product2/1
  Product2/1 -> d_min/1
  BC/1 -> bus1/1
  Switch/1 -> Sum1/2, Mux2/4  "Pt"
  BS1/4 -> Switch/3  "<Pt>"
  Pt_new/1 -> Switch/1
  Switch1/1 -> Mux2/6
  BS2/6 -> Switch1/3  "<Palv>"
  BS2/3 -> Switch/2, Switch1/2  "<while>"
  BS2/5 -> Switch1/1  "<Palv_next>"
  In2/1 -> BS2/1
  BS2/1 -> Mux2/2  "<rate_asc>"

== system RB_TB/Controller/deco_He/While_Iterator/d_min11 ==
  note: Model: RB_TB/Controller/deco_He/While_Iterator/d_minX
  Pt_new : Inport  Port=1  LatchInput=off
  In1 : Inport  Port=2  LatchInput=off
  In2 : Inport  Port=3  LatchInput=off
  BC : BusCreator  DialogController=Simulink.DDGSource_Bus
  BS1 : BusSelector  DialogController=Simulink.DDGSource_Bus  OutputSignals=He_b,M0,He_k,Pt
  BS2 : BusSelector  DialogController=Simulink.DDGSource_Bus  OutputSignals=rate_asc,asc_time,while,cnc_He,Palv_next,Palv
  Mux2 : Mux  Inputs=6
  Product2 : Product
  Sum1 : Sum  Inputs=-+|
  Switch : Switch  Threshold=2
  Switch1 : Switch  Threshold=2
  fnc : Fcn  Expr=u(6)-u(5)*u(2)*(u(3)-1/u(1))-(u(6)-u(4)+u(5)*u(2)/u(1))*exp(-u(1)*u(3))
  prod : Gain  Gain=10
  bus1 : Outport
  d_min : Outport  Port=2
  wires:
  BS2/1 -> Mux2/2  "<rate_asc>"
  In2/1 -> BS2/1
  BS2/5 -> Switch1/1  "<Palv_next>"
  BS2/3 -> Switch1/2, Switch/2  "<while>"
  BS2/6 -> Switch1/3  "<Palv>"
  Switch1/1 -> Mux2/6
  Pt_new/1 -> Switch/1
  BS1/4 -> Switch/3  "<Pt>"
  Switch/1 -> Mux2/4, Sum1/2  "Pt"
  BC/1 -> bus1/1
  Product2/1 -> d_min/1
  prod/1 -> Product2/1
  Sum1/1 -> Product2/2
  In1/1 -> BS1/1
  BS2/4 -> Mux2/5  "<cnc_He>"
  BS2/2 -> Mux2/3  "<asc_time>"
  fnc/1 -> BC/4  "Pt_stop"
  Mux2/1 -> fnc/1
  BS1/2 -> BC/2, Sum1/1  "<M0>"
  BS1/1 -> BC/1, prod/1  "<He_b>"
  BS1/3 -> BC/3, Mux2/1  "<He_k>"

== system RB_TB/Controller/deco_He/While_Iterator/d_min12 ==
  note: Model: RB_TB/Controller/deco_He/While_Iterator/d_minX
  Pt_new : Inport  Port=1  LatchInput=off
  In1 : Inport  Port=2  LatchInput=off
  In2 : Inport  Port=3  LatchInput=off
  BC : BusCreator  DialogController=Simulink.DDGSource_Bus
  BS1 : BusSelector  DialogController=Simulink.DDGSource_Bus  OutputSignals=He_b,M0,He_k,Pt
  BS2 : BusSelector  DialogController=Simulink.DDGSource_Bus  OutputSignals=rate_asc,asc_time,while,cnc_He,Palv_next,Palv
  Mux2 : Mux  Inputs=6
  Product2 : Product
  Sum1 : Sum  Inputs=-+|
  Switch : Switch  Threshold=2
  Switch1 : Switch  Threshold=2
  fnc : Fcn  Expr=u(6)-u(5)*u(2)*(u(3)-1/u(1))-(u(6)-u(4)+u(5)*u(2)/u(1))*exp(-u(1)*u(3))
  prod : Gain  Gain=10
  bus1 : Outport
  d_min : Outport  Port=2
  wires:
  BS1/3 -> Mux2/1, BC/3  "<He_k>"
  BS1/1 -> prod/1, BC/1  "<He_b>"
  BS1/2 -> Sum1/1, BC/2  "<M0>"
  Mux2/1 -> fnc/1
  fnc/1 -> BC/4  "Pt_stop"
  BS2/2 -> Mux2/3  "<asc_time>"
  BS2/4 -> Mux2/5  "<cnc_He>"
  In1/1 -> BS1/1
  Sum1/1 -> Product2/2
  prod/1 -> Product2/1
  Product2/1 -> d_min/1
  BC/1 -> bus1/1
  Switch/1 -> Sum1/2, Mux2/4  "Pt"
  BS1/4 -> Switch/3  "<Pt>"
  Pt_new/1 -> Switch/1
  Switch1/1 -> Mux2/6
  BS2/6 -> Switch1/3  "<Palv>"
  BS2/3 -> Switch/2, Switch1/2  "<while>"
  BS2/5 -> Switch1/1  "<Palv_next>"
  In2/1 -> BS2/1
  BS2/1 -> Mux2/2  "<rate_asc>"

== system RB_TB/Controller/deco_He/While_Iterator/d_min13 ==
  note: Model: RB_TB/Controller/deco_He/While_Iterator/d_minX
  Pt_new : Inport  Port=1  LatchInput=off
  In1 : Inport  Port=2  LatchInput=off
  In2 : Inport  Port=3  LatchInput=off
  BC : BusCreator  DialogController=Simulink.DDGSource_Bus
  BS1 : BusSelector  DialogController=Simulink.DDGSource_Bus  OutputSignals=He_b,M0,He_k,Pt
  BS2 : BusSelector  DialogController=Simulink.DDGSource_Bus  OutputSignals=rate_asc,asc_time,while,cnc_He,Palv_next,Palv
  Mux2 : Mux  Inputs=6
  Product2 : Product
  Sum1 : Sum  Inputs=-+|
  Switch : Switch  Threshold=2
  Switch1 : Switch  Threshold=2
  fnc : Fcn  Expr=u(6)-u(5)*u(2)*(u(3)-1/u(1))-(u(6)-u(4)+u(5)*u(2)/u(1))*exp(-u(1)*u(3))
  prod : Gain  Gain=10
  bus1 : Outport
  d_min : Outport  Port=2
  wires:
  BS2/1 -> Mux2/2  "<rate_asc>"
  In2/1 -> BS2/1
  BS2/5 -> Switch1/1  "<Palv_next>"
  BS2/3 -> Switch1/2, Switch/2  "<while>"
  BS2/6 -> Switch1/3  "<Palv>"
  Switch1/1 -> Mux2/6
  Pt_new/1 -> Switch/1
  BS1/4 -> Switch/3  "<Pt>"
  Switch/1 -> Mux2/4, Sum1/2  "Pt"
  BC/1 -> bus1/1
  Product2/1 -> d_min/1
  prod/1 -> Product2/1
  Sum1/1 -> Product2/2
  In1/1 -> BS1/1
  BS2/4 -> Mux2/5  "<cnc_He>"
  BS2/2 -> Mux2/3  "<asc_time>"
  fnc/1 -> BC/4  "Pt_stop"
  Mux2/1 -> fnc/1
  BS1/2 -> BC/2, Sum1/1  "<M0>"
  BS1/1 -> BC/1, prod/1  "<He_b>"
  BS1/3 -> BC/3, Mux2/1  "<He_k>"

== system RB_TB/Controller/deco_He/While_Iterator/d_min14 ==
  note: Model: RB_TB/Controller/deco_He/While_Iterator/d_minX
  Pt_new : Inport  Port=1  LatchInput=off
  In1 : Inport  Port=2  LatchInput=off
  In2 : Inport  Port=3  LatchInput=off
  BC : BusCreator  DialogController=Simulink.DDGSource_Bus
  BS1 : BusSelector  DialogController=Simulink.DDGSource_Bus  OutputSignals=He_b,M0,He_k,Pt
  BS2 : BusSelector  DialogController=Simulink.DDGSource_Bus  OutputSignals=rate_asc,asc_time,while,cnc_He,Palv_next,Palv
  Mux2 : Mux  Inputs=6
  Product2 : Product
  Sum1 : Sum  Inputs=-+|
  Switch : Switch  Threshold=2
  Switch1 : Switch  Threshold=2
  fnc : Fcn  Expr=u(6)-u(5)*u(2)*(u(3)-1/u(1))-(u(6)-u(4)+u(5)*u(2)/u(1))*exp(-u(1)*u(3))
  prod : Gain  Gain=10
  bus1 : Outport
  d_min : Outport  Port=2
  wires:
  BS1/3 -> Mux2/1, BC/3  "<He_k>"
  BS1/1 -> prod/1, BC/1  "<He_b>"
  BS1/2 -> Sum1/1, BC/2  "<M0>"
  Mux2/1 -> fnc/1
  fnc/1 -> BC/4  "Pt_stop"
  BS2/2 -> Mux2/3  "<asc_time>"
  BS2/4 -> Mux2/5  "<cnc_He>"
  In1/1 -> BS1/1
  Sum1/1 -> Product2/2
  prod/1 -> Product2/1
  Product2/1 -> d_min/1
  BC/1 -> bus1/1
  Switch/1 -> Sum1/2, Mux2/4  "Pt"
  BS1/4 -> Switch/3  "<Pt>"
  Pt_new/1 -> Switch/1
  Switch1/1 -> Mux2/6
  BS2/6 -> Switch1/3  "<Palv>"
  BS2/3 -> Switch/2, Switch1/2  "<while>"
  BS2/5 -> Switch1/1  "<Palv_next>"
  In2/1 -> BS2/1
  BS2/1 -> Mux2/2  "<rate_asc>"

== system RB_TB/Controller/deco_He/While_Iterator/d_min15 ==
  note: Model: RB_TB/Controller/deco_He/While_Iterator/d_minX
  Pt_new : Inport  Port=1  LatchInput=off
  In1 : Inport  Port=2  LatchInput=off
  In2 : Inport  Port=3  LatchInput=off
  BC : BusCreator  DialogController=Simulink.DDGSource_Bus
  BS1 : BusSelector  DialogController=Simulink.DDGSource_Bus  OutputSignals=He_b,M0,He_k,Pt
  BS2 : BusSelector  DialogController=Simulink.DDGSource_Bus  OutputSignals=rate_asc,asc_time,while,cnc_He,Palv_next,Palv
  Mux2 : Mux  Inputs=6
  Product2 : Product
  Sum1 : Sum  Inputs=-+|
  Switch : Switch  Threshold=2
  Switch1 : Switch  Threshold=2
  fnc : Fcn  Expr=u(6)-u(5)*u(2)*(u(3)-1/u(1))-(u(6)-u(4)+u(5)*u(2)/u(1))*exp(-u(1)*u(3))
  prod : Gain  Gain=10
  bus1 : Outport
  d_min : Outport  Port=2
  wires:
  BS2/1 -> Mux2/2  "<rate_asc>"
  In2/1 -> BS2/1
  BS2/5 -> Switch1/1  "<Palv_next>"
  BS2/3 -> Switch1/2, Switch/2  "<while>"
  BS2/6 -> Switch1/3  "<Palv>"
  Switch1/1 -> Mux2/6
  Pt_new/1 -> Switch/1
  BS1/4 -> Switch/3  "<Pt>"
  Switch/1 -> Mux2/4, Sum1/2  "Pt"
  BC/1 -> bus1/1
  Product2/1 -> d_min/1
  prod/1 -> Product2/1
  Sum1/1 -> Product2/2
  In1/1 -> BS1/1
  BS2/4 -> Mux2/5  "<cnc_He>"
  BS2/2 -> Mux2/3  "<asc_time>"
  fnc/1 -> BC/4  "Pt_stop"
  Mux2/1 -> fnc/1
  BS1/2 -> BC/2, Sum1/1  "<M0>"
  BS1/1 -> BC/1, prod/1  "<He_b>"
  BS1/3 -> BC/3, Mux2/1  "<He_k>"

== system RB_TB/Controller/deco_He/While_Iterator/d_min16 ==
  note: Model: RB_TB/Controller/deco_He/While_Iterator/d_minX
  Pt_new : Inport  Port=1  LatchInput=off
  In1 : Inport  Port=2  LatchInput=off
  In2 : Inport  Port=3  LatchInput=off
  BC : BusCreator  DialogController=Simulink.DDGSource_Bus
  BS1 : BusSelector  DialogController=Simulink.DDGSource_Bus  OutputSignals=He_b,M0,He_k,Pt
  BS2 : BusSelector  DialogController=Simulink.DDGSource_Bus  OutputSignals=rate_asc,asc_time,while,cnc_He,Palv_next,Palv
  Mux2 : Mux  Inputs=6
  Product2 : Product
  Sum1 : Sum  Inputs=-+|
  Switch : Switch  Threshold=2
  Switch1 : Switch  Threshold=2
  fnc : Fcn  Expr=u(6)-u(5)*u(2)*(u(3)-1/u(1))-(u(6)-u(4)+u(5)*u(2)/u(1))*exp(-u(1)*u(3))
  prod : Gain  Gain=10
  bus1 : Outport
  d_min : Outport  Port=2
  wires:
  BS1/3 -> Mux2/1, BC/3  "<He_k>"
  BS1/1 -> prod/1, BC/1  "<He_b>"
  BS1/2 -> Sum1/1, BC/2  "<M0>"
  Mux2/1 -> fnc/1
  fnc/1 -> BC/4  "Pt_stop"
  BS2/2 -> Mux2/3  "<asc_time>"
  BS2/4 -> Mux2/5  "<cnc_He>"
  In1/1 -> BS1/1
  Sum1/1 -> Product2/2
  prod/1 -> Product2/1
  Product2/1 -> d_min/1
  BC/1 -> bus1/1
  Switch/1 -> Sum1/2, Mux2/4  "Pt"
  BS1/4 -> Switch/3  "<Pt>"
  Pt_new/1 -> Switch/1
  Switch1/1 -> Mux2/6
  BS2/6 -> Switch1/3  "<Palv>"
  BS2/3 -> Switch/2, Switch1/2  "<while>"
  BS2/5 -> Switch1/1  "<Palv_next>"
  In2/1 -> BS2/1
  BS2/1 -> Mux2/2  "<rate_asc>"

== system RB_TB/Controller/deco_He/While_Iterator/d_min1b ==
  note: Model: RB_TB/Controller/deco_He/While_Iterator/d_minX
  Pt_new : Inport  Port=1  LatchInput=off
  In1 : Inport  Port=2  LatchInput=off
  In2 : Inport  Port=3  LatchInput=off
  BC : BusCreator  DialogController=Simulink.DDGSource_Bus
  BS1 : BusSelector  DialogController=Simulink.DDGSource_Bus  OutputSignals=He_b,M0,He_k,Pt
  BS2 : BusSelector  DialogController=Simulink.DDGSource_Bus  OutputSignals=rate_asc,asc_time,while,cnc_He,Palv_next,Palv
  Mux2 : Mux  Inputs=6
  Product2 : Product
  Sum1 : Sum  Inputs=-+|
  Switch : Switch  Threshold=2
  Switch1 : Switch  Threshold=2
  fnc : Fcn  Expr=u(6)-u(5)*u(2)*(u(3)-1/u(1))-(u(6)-u(4)+u(5)*u(2)/u(1))*exp(-u(1)*u(3))
  prod : Gain  Gain=10
  bus1 : Outport
  d_min : Outport  Port=2
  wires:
  BS2/1 -> Mux2/2  "<rate_asc>"
  In2/1 -> BS2/1
  BS2/5 -> Switch1/1  "<Palv_next>"
  BS2/3 -> Switch1/2, Switch/2  "<while>"
  BS2/6 -> Switch1/3  "<Palv>"
  Switch1/1 -> Mux2/6
  Pt_new/1 -> Switch/1
  BS1/4 -> Switch/3  "<Pt>"
  Switch/1 -> Mux2/4, Sum1/2  "Pt"
  BC/1 -> bus1/1
  Product2/1 -> d_min/1
  prod/1 -> Product2/1
  Sum1/1 -> Product2/2
  In1/1 -> BS1/1
  BS2/4 -> Mux2/5  "<cnc_He>"
  BS2/2 -> Mux2/3  "<asc_time>"
  fnc/1 -> BC/4  "Pt_stop"
  Mux2/1 -> fnc/1
  BS1/2 -> BC/2, Sum1/1  "<M0>"
  BS1/1 -> BC/1, prod/1  "<He_b>"
  BS1/3 -> BC/3, Mux2/1  "<He_k>"

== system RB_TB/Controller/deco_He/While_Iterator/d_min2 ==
  note: Model: RB_TB/Controller/deco_He/While_Iterator/d_minX
  Pt_new : Inport  Port=1  LatchInput=off
  In1 : Inport  Port=2  LatchInput=off
  In2 : Inport  Port=3  LatchInput=off
  BC : BusCreator  DialogController=Simulink.DDGSource_Bus
  BS1 : BusSelector  DialogController=Simulink.DDGSource_Bus  OutputSignals=He_b,M0,He_k,Pt
  BS2 : BusSelector  DialogController=Simulink.DDGSource_Bus  OutputSignals=rate_asc,asc_time,while,cnc_He,Palv_next,Palv
  Mux2 : Mux  Inputs=6
  Product2 : Product
  Sum1 : Sum  Inputs=-+|
  Switch : Switch  Threshold=2
  Switch1 : Switch  Threshold=2
  fnc : Fcn  Expr=u(6)-u(5)*u(2)*(u(3)-1/u(1))-(u(6)-u(4)+u(5)*u(2)/u(1))*exp(-u(1)*u(3))
  prod : Gain  Gain=10
  bus1 : Outport
  d_min : Outport  Port=2
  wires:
  BS1/3 -> Mux2/1, BC/3  "<He_k>"
  BS1/1 -> prod/1, BC/1  "<He_b>"
  BS1/2 -> Sum1/1, BC/2  "<M0>"
  Mux2/1 -> fnc/1
  fnc/1 -> BC/4  "Pt_stop"
  BS2/2 -> Mux2/3  "<asc_time>"
  BS2/4 -> Mux2/5  "<cnc_He>"
  In1/1 -> BS1/1
  Sum1/1 -> Product2/2
  prod/1 -> Product2/1
  Product2/1 -> d_min/1
  BC/1 -> bus1/1
  Switch/1 -> Sum1/2, Mux2/4  "Pt"
  BS1/4 -> Switch/3  "<Pt>"
  Pt_new/1 -> Switch/1
  Switch1/1 -> Mux2/6
  BS2/6 -> Switch1/3  "<Palv>"
  BS2/3 -> Switch/2, Switch1/2  "<while>"
  BS2/5 -> Switch1/1  "<Palv_next>"
  In2/1 -> BS2/1
  BS2/1 -> Mux2/2  "<rate_asc>"

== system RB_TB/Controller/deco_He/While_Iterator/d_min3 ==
  note: Model: RB_TB/Controller/deco_He/While_Iterator/d_minX
  Pt_new : Inport  Port=1  LatchInput=off
  In1 : Inport  Port=2  LatchInput=off
  In2 : Inport  Port=3  LatchInput=off
  BC : BusCreator  DialogController=Simulink.DDGSource_Bus
  BS1 : BusSelector  DialogController=Simulink.DDGSource_Bus  OutputSignals=He_b,M0,He_k,Pt
  BS2 : BusSelector  DialogController=Simulink.DDGSource_Bus  OutputSignals=rate_asc,asc_time,while,cnc_He,Palv_next,Palv
  Mux2 : Mux  Inputs=6
  Product2 : Product
  Sum1 : Sum  Inputs=-+|
  Switch : Switch  Threshold=2
  Switch1 : Switch  Threshold=2
  fnc : Fcn  Expr=u(6)-u(5)*u(2)*(u(3)-1/u(1))-(u(6)-u(4)+u(5)*u(2)/u(1))*exp(-u(1)*u(3))
  prod : Gain  Gain=10
  bus1 : Outport
  d_min : Outport  Port=2
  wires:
  BS2/1 -> Mux2/2  "<rate_asc>"
  In2/1 -> BS2/1
  BS2/5 -> Switch1/1  "<Palv_next>"
  BS2/3 -> Switch1/2, Switch/2  "<while>"
  BS2/6 -> Switch1/3  "<Palv>"
  Switch1/1 -> Mux2/6
  Pt_new/1 -> Switch/1
  BS1/4 -> Switch/3  "<Pt>"
  Switch/1 -> Mux2/4, Sum1/2  "Pt"
  BC/1 -> bus1/1
  Product2/1 -> d_min/1
  prod/1 -> Product2/1
  Sum1/1 -> Product2/2
  In1/1 -> BS1/1
  BS2/4 -> Mux2/5  "<cnc_He>"
  BS2/2 -> Mux2/3  "<asc_time>"
  fnc/1 -> BC/4  "Pt_stop"
  Mux2/1 -> fnc/1
  BS1/2 -> BC/2, Sum1/1  "<M0>"
  BS1/1 -> BC/1, prod/1  "<He_b>"
  BS1/3 -> BC/3, Mux2/1  "<He_k>"

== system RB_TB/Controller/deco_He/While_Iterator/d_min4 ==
  note: Model: RB_TB/Controller/deco_He/While_Iterator/d_minX
  Pt_new : Inport  Port=1  LatchInput=off
  In1 : Inport  Port=2  LatchInput=off
  In2 : Inport  Port=3  LatchInput=off
  BC : BusCreator  DialogController=Simulink.DDGSource_Bus
  BS1 : BusSelector  DialogController=Simulink.DDGSource_Bus  OutputSignals=He_b,M0,He_k,Pt
  BS2 : BusSelector  DialogController=Simulink.DDGSource_Bus  OutputSignals=rate_asc,asc_time,while,cnc_He,Palv_next,Palv
  Mux2 : Mux  Inputs=6
  Product2 : Product
  Sum1 : Sum  Inputs=-+|
  Switch : Switch  Threshold=2
  Switch1 : Switch  Threshold=2
  fnc : Fcn  Expr=u(6)-u(5)*u(2)*(u(3)-1/u(1))-(u(6)-u(4)+u(5)*u(2)/u(1))*exp(-u(1)*u(3))
  prod : Gain  Gain=10
  bus1 : Outport
  d_min : Outport  Port=2
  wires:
  BS1/3 -> Mux2/1, BC/3  "<He_k>"
  BS1/1 -> prod/1, BC/1  "<He_b>"
  BS1/2 -> Sum1/1, BC/2  "<M0>"
  Mux2/1 -> fnc/1
  fnc/1 -> BC/4  "Pt_stop"
  BS2/2 -> Mux2/3  "<asc_time>"
  BS2/4 -> Mux2/5  "<cnc_He>"
  In1/1 -> BS1/1
  Sum1/1 -> Product2/2
  prod/1 -> Product2/1
  Product2/1 -> d_min/1
  BC/1 -> bus1/1
  Switch/1 -> Sum1/2, Mux2/4  "Pt"
  BS1/4 -> Switch/3  "<Pt>"
  Pt_new/1 -> Switch/1
  Switch1/1 -> Mux2/6
  BS2/6 -> Switch1/3  "<Palv>"
  BS2/3 -> Switch/2, Switch1/2  "<while>"
  BS2/5 -> Switch1/1  "<Palv_next>"
  In2/1 -> BS2/1
  BS2/1 -> Mux2/2  "<rate_asc>"

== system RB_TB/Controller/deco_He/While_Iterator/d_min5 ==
  note: Model: RB_TB/Controller/deco_He/While_Iterator/d_minX
  Pt_new : Inport  Port=1  LatchInput=off
  In1 : Inport  Port=2  LatchInput=off
  In2 : Inport  Port=3  LatchInput=off
  BC : BusCreator  DialogController=Simulink.DDGSource_Bus
  BS1 : BusSelector  DialogController=Simulink.DDGSource_Bus  OutputSignals=He_b,M0,He_k,Pt
  BS2 : BusSelector  DialogController=Simulink.DDGSource_Bus  OutputSignals=rate_asc,asc_time,while,cnc_He,Palv_next,Palv
  Mux2 : Mux  Inputs=6
  Product2 : Product
  Sum1 : Sum  Inputs=-+|
  Switch : Switch  Threshold=2
  Switch1 : Switch  Threshold=2
  fnc : Fcn  Expr=u(6)-u(5)*u(2)*(u(3)-1/u(1))-(u(6)-u(4)+u(5)*u(2)/u(1))*exp(-u(1)*u(3))
  prod : Gain  Gain=10
  bus1 : Outport
  d_min : Outport  Port=2
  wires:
  BS2/1 -> Mux2/2  "<rate_asc>"
  In2/1 -> BS2/1
  BS2/5 -> Switch1/1  "<Palv_next>"
  BS2/3 -> Switch1/2, Switch/2  "<while>"
  BS2/6 -> Switch1/3  "<Palv>"
  Switch1/1 -> Mux2/6
  Pt_new/1 -> Switch/1
  BS1/4 -> Switch/3  "<Pt>"
  Switch/1 -> Mux2/4, Sum1/2  "Pt"
  BC/1 -> bus1/1
  Product2/1 -> d_min/1
  prod/1 -> Product2/1
  Sum1/1 -> Product2/2
  In1/1 -> BS1/1
  BS2/4 -> Mux2/5  "<cnc_He>"
  BS2/2 -> Mux2/3  "<asc_time>"
  fnc/1 -> BC/4  "Pt_stop"
  Mux2/1 -> fnc/1
  BS1/2 -> BC/2, Sum1/1  "<M0>"
  BS1/1 -> BC/1, prod/1  "<He_b>"
  BS1/3 -> BC/3, Mux2/1  "<He_k>"

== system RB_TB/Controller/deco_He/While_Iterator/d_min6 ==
  note: Model: RB_TB/Controller/deco_He/While_Iterator/d_minX
  Pt_new : Inport  Port=1  LatchInput=off
  In1 : Inport  Port=2  LatchInput=off
  In2 : Inport  Port=3  LatchInput=off
  BC : BusCreator  DialogController=Simulink.DDGSource_Bus
  BS1 : BusSelector  DialogController=Simulink.DDGSource_Bus  OutputSignals=He_b,M0,He_k,Pt
  BS2 : BusSelector  DialogController=Simulink.DDGSource_Bus  OutputSignals=rate_asc,asc_time,while,cnc_He,Palv_next,Palv
  Mux2 : Mux  Inputs=6
  Product2 : Product
  Sum1 : Sum  Inputs=-+|
  Switch : Switch  Threshold=2
  Switch1 : Switch  Threshold=2
  fnc : Fcn  Expr=u(6)-u(5)*u(2)*(u(3)-1/u(1))-(u(6)-u(4)+u(5)*u(2)/u(1))*exp(-u(1)*u(3))
  prod : Gain  Gain=10
  bus1 : Outport
  d_min : Outport  Port=2
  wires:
  BS1/3 -> Mux2/1, BC/3  "<He_k>"
  BS1/1 -> prod/1, BC/1  "<He_b>"
  BS1/2 -> Sum1/1, BC/2  "<M0>"
  Mux2/1 -> fnc/1
  fnc/1 -> BC/4  "Pt_stop"
  BS2/2 -> Mux2/3  "<asc_time>"
  BS2/4 -> Mux2/5  "<cnc_He>"
  In1/1 -> BS1/1
  Sum1/1 -> Product2/2
  prod/1 -> Product2/1
  Product2/1 -> d_min/1
  BC/1 -> bus1/1
  Switch/1 -> Sum1/2, Mux2/4  "Pt"
  BS1/4 -> Switch/3  "<Pt>"
  Pt_new/1 -> Switch/1
  Switch1/1 -> Mux2/6
  BS2/6 -> Switch1/3  "<Palv>"
  BS2/3 -> Switch/2, Switch1/2  "<while>"
  BS2/5 -> Switch1/1  "<Palv_next>"
  In2/1 -> BS2/1
  BS2/1 -> Mux2/2  "<rate_asc>"

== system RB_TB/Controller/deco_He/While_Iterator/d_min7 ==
  note: Model: RB_TB/Controller/deco_He/While_Iterator/d_minX
  Pt_new : Inport  Port=1  LatchInput=off
  In1 : Inport  Port=2  LatchInput=off
  In2 : Inport  Port=3  LatchInput=off
  BC : BusCreator  DialogController=Simulink.DDGSource_Bus
  BS1 : BusSelector  DialogController=Simulink.DDGSource_Bus  OutputSignals=He_b,M0,He_k,Pt
  BS2 : BusSelector  DialogController=Simulink.DDGSource_Bus  OutputSignals=rate_asc,asc_time,while,cnc_He,Palv_next,Palv
  Mux2 : Mux  Inputs=6
  Product2 : Product
  Sum1 : Sum  Inputs=-+|
  Switch : Switch  Threshold=2
  Switch1 : Switch  Threshold=2
  fnc : Fcn  Expr=u(6)-u(5)*u(2)*(u(3)-1/u(1))-(u(6)-u(4)+u(5)*u(2)/u(1))*exp(-u(1)*u(3))
  prod : Gain  Gain=10
  bus1 : Outport
  d_min : Outport  Port=2
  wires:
  BS2/1 -> Mux2/2  "<rate_asc>"
  In2/1 -> BS2/1
  BS2/5 -> Switch1/1  "<Palv_next>"
  BS2/3 -> Switch1/2, Switch/2  "<while>"
  BS2/6 -> Switch1/3  "<Palv>"
  Switch1/1 -> Mux2/6
  Pt_new/1 -> Switch/1
  BS1/4 -> Switch/3  "<Pt>"
  Switch/1 -> Mux2/4, Sum1/2  "Pt"
  BC/1 -> bus1/1
  Product2/1 -> d_min/1
  prod/1 -> Product2/1
  Sum1/1 -> Product2/2
  In1/1 -> BS1/1
  BS2/4 -> Mux2/5  "<cnc_He>"
  BS2/2 -> Mux2/3  "<asc_time>"
  fnc/1 -> BC/4  "Pt_stop"
  Mux2/1 -> fnc/1
  BS1/2 -> BC/2, Sum1/1  "<M0>"
  BS1/1 -> BC/1, prod/1  "<He_b>"
  BS1/3 -> BC/3, Mux2/1  "<He_k>"
